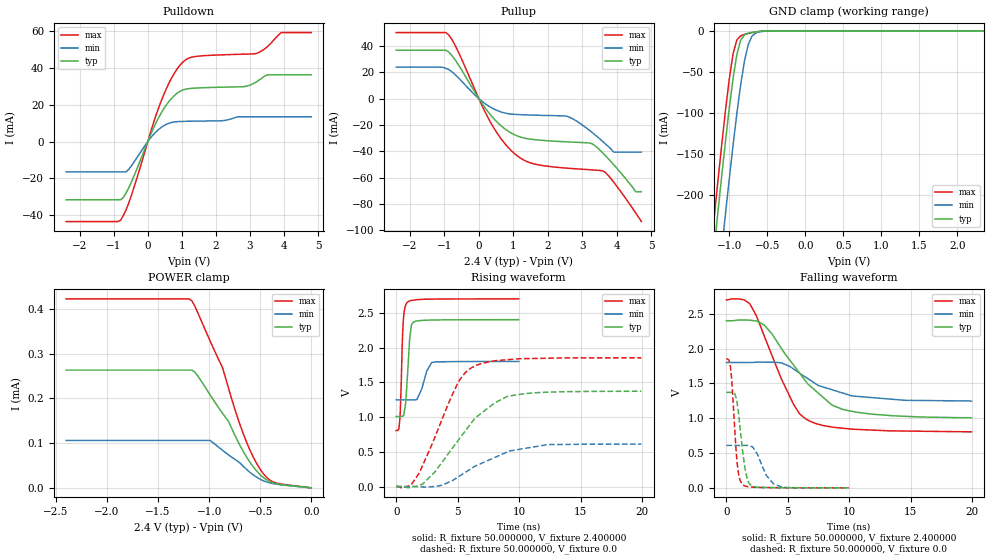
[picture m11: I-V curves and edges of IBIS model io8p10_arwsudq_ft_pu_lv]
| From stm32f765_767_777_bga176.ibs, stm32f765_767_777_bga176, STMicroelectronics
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|   Model io8p10_arwsudq_ft_pu_lv
[Model]  io8p10_arwsudq_ft_pu_lv
Model_type I/O
Polarity   Non-Inverting
Enable   Active-Low
Vinl =   0.720000V
Vinh =   1.680000V
Vmeas =  1.200000V
Cref =   40.000000pF
Rref =   100.000000M
Vref =   0.0V
C_comp   2.828000pF   2.774700pF   2.917100pF
[Temperature Range]   25.000000   0.125000k   -40.000000
[Pullup Reference]   2.400000V   1.800000V   2.700000V
[Pulldown Reference]   0.0V   0.0V   0.0V
[POWER Clamp Reference]   2.400000V   1.800000V   2.700000V
[GND Clamp Reference]   0.0V   0.0V   0.0V
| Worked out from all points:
|   slope of the pulldown table from 0 to 0.36 V, typ, clamps not added: 25 ohm
|   slope of the pullup table from 0 to 0.36 V, typ, clamps not added: 27.7 ohm
|   GND clamp passes 1 mA (typ) near -0.62 V on its own axis
|   rising waveform, R_fixture 50.000000, V_fixture 2.400000: 20-80 % time 291ps typ, 616ps min, 205ps max; typ from 1.01 V to 2.4 V
|   rising waveform, R_fixture 50.000000, V_fixture 0.0: 20-80 % time 3.81ns typ, 4.01ns min, 2.68ns max; typ from 0.001 V to 1.37 V
|   falling waveform, R_fixture 50.000000, V_fixture 2.400000: 20-80 % time 3.92ns typ, 3.92ns min, 2.75ns max; typ from 2.4 V to 1.01 V
|   falling waveform, R_fixture 50.000000, V_fixture 0.0: 20-80 % time 548ps typ, 1.01ns min, 410ps max; typ from 1.37 V to 0.001 V
[Pulldown]
|Voltage   I(typ)   I(min)   I(max)
-2.4V     -31.67mA   -16.51mA   -43.52mA
-800mV    -31.67mA   -16.51mA   -42.87mA
-480mV    -21.98mA   -13.17mA   -29.21mA
80mV      3.63mA     1.966mA    5.012mA
480mV     18.16mA    8.738mA    26.02mA
800mV     25.38mA    10.72mA    37.77mA
1.12V     28.53mA    11.02mA    44.6mA
2.8V      29.84mA    13.46mA    47.53mA
3.2V      32.6mA     13.46mA    48.03mA
3.52V     36.31mA    13.46mA    51.75mA
3.92V     36.31mA    13.46mA    59.29mA
4.8V      36.31mA    13.46mA    59.29mA
[Pullup]
|Voltage   I(typ)   I(min)   I(max)
-2.4V     36.83mA    24.03mA    50.23mA
-960mV    36.83mA    23.01mA    50.23mA
-640mV    27.62mA    17.03mA    37.94mA
320mV     -11.75mA   -6.207mA   -17.08mA
960mV     -26.47mA   -11.82mA   -40.02mA
1.52V     -30.88mA   -12.51mA   -49.05mA
2.56V     -32.88mA   -13.48mA   -52.9mA
3.28V     -34.19mA   -25.52mA   -54.17mA
3.6V      -41.32mA   -32.62mA   -54.98mA
3.92V     -50.33mA   -40.7mA    -63.65mA
4.56V     -70.9mA    -40.7mA    -87.11mA
4.72V     -70.9mA    -40.7mA    -93.5mA
[GND_clamp]
|Voltage   I(typ)   I(min)   I(max)
-2.4V     -1.425A    -1.509A    -1.395A
-1.25V    -311.8mA   -402mA     -274.5mA
-1.2V     -266mA     -356.2mA   -228.4mA
-1.15V    -220.9mA   -310.9mA   -183.1mA
-1.1V     -176.9mA   -266.3mA   -139mA
-1.05V    -134.3mA   -222.6mA   -97.01mA
-950mV    -57.81mA   -139.1mA   -27.86mA
-900mV    -28.73mA   -100.5mA   -11.04mA
-850mV    -11.29mA   -65.69mA   -6.054mA
-750mV    -2.852mA   -16.6mA    -3.179mA
-600mV    -750uA     -1.167mA   -738.5uA
2.35V     0A         0A         0A
[POWER_clamp]
|Voltage   I(typ)   I(min)   I(max)
-2.4V     263.2uA    106uA      422.4uA
-1.17V    263.2uA    106uA      418.5uA
-1.11V    250.1uA    106uA      391.1uA
-990mV    207.7uA    106uA      328.2uA
-870mV    167.2uA    84.17uA    269.6uA
-810mV    148.5uA    73.71uA    222.7uA
-660mV    79.21uA    47.09uA    117.6uA
-570mV    47.82uA    29.3uA     69.9uA
-510mV    31.66uA    20.4uA     45.18uA
-420mV    15.55uA    11.87uA    19.89uA
-360mV    10.34uA    8.845uA    12.09uA
0V        0A         0A         0A
[Ramp]
| variable   typ   min   max
dV/dt_r  0.82201/3.80878n   0.36592/4.01030n   1.11124/2.67502n
dV/dt_f  0.83274/3.92665n   0.33240/3.96864n   1.13569/2.74622n
R_load = 50.000000
[Rising Waveform]
R_fixture= 50.000000
V_fixture= 2.400000
V_fixture_min= 1.800000
V_fixture_max= 2.700000
|time   V(typ)   V(min)   V(max)
0s        1.007V     1.247V     805.7mV
220.2ps   1.007V     1.247V     831.4mV
300.3ps   1.007V     1.247V     976.8mV
560.6ps   1.017V     1.247V     2.338V
780.8ps   1.22V      1.247V     2.614V
880.9ps   1.501V     1.247V     2.645V
1.101ns   2.136V     1.247V     2.67V
1.461ns   2.371V     1.247V     2.683V
2.903ns   2.395V     1.784V     2.696V
9.97ns    2.4V       1.8V       2.699V
[Rising Waveform]
R_fixture= 50.000000
V_fixture= 0.0
V_fixture_min= 0.0
V_fixture_max= 0.0
|time   V(typ)   V(min)   V(max)
0s        1.051mV    906.3uV    1.513mV
1.241ns   -6.967mV   1.019mV    30.63mV
1.882ns   18.56mV    -2.335mV   198.6mV
3.163ns   213.4mV    2.019mV    718.3mV
5.005ns   656.4mV    134.6mV    1.486V
6.246ns   946.4mV    275.6mV    1.721V
7.968ns   1.198V     414.6mV    1.808V
9.249ns   1.303V     512.8mV    1.828V
12.33ns   1.358V     603.5mV    1.846V
19.94ns   1.371V     610.2mV    1.852V
[Falling Waveform]
R_fixture= 50.000000
V_fixture= 2.400000
V_fixture_min= 1.800000
V_fixture_max= 2.700000
|time   V(typ)   V(min)   V(max)
0s        2.4V       1.8V       2.699V
1.441ns   2.41V      1.8V       2.7V
1.922ns   2.407V     1.801V     2.64V
3.083ns   2.338V     1.805V     2.182V
4.484ns   2.001V     1.795V     1.563V
5.445ns   1.768V     1.71V      1.207V
6.607ns   1.496V     1.571V     974.8mV
8.569ns   1.192V     1.411V     874.6mV
9.85ns    1.111V     1.34V      849.9mV
19.94ns   1.007V     1.247V     805.7mV
[Falling Waveform]
R_fixture= 50.000000
V_fixture= 0.0
V_fixture_min= 0.0
V_fixture_max= 0.0
|time   V(typ)   V(min)   V(max)
0s        1.371V     610.2mV    1.852V
340.3ps   1.371V     610.2mV    1.729V
440.4ps   1.371V     610.2mV    1.542V
840.8ps   1.262V     610mV      439.8mV
1.041ns   990.4mV    609.7mV    158.2mV
1.321ns   531.5mV    609.9mV    50.78mV
1.702ns   127.8mV    610.7mV    18.38mV
2.182ns   22.8mV     579.3mV    9.573mV
3.844ns   4.273mV    58.3mV     3.634mV
9.97ns    1.051mV    906.3uV    1.513mV
